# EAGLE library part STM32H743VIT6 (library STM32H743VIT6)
ARM Microcontrollers - MCU High-performance and DSP with DP-FPU, ARM Cortex-M7 MCU with 2MBytes Flash, 1MB RAM, 400 MHz CPU, Art Accelerator, L1 cache, external memory interface, large set of peripherals Source: Datasheet
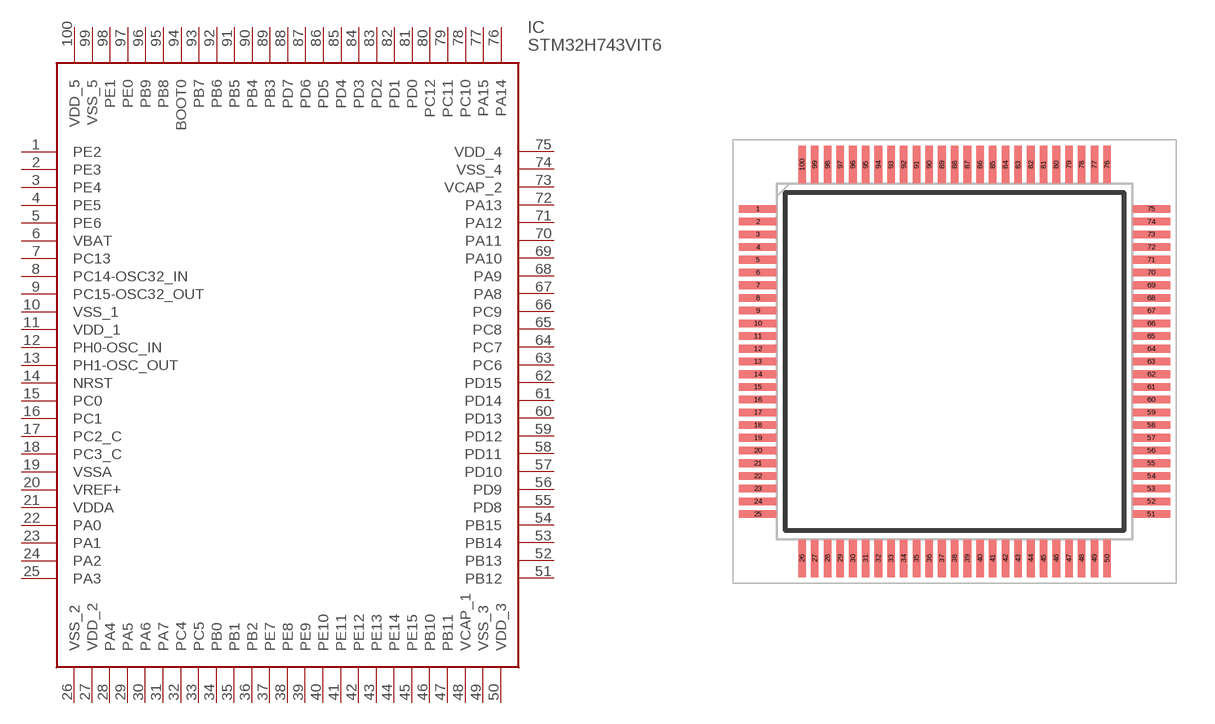
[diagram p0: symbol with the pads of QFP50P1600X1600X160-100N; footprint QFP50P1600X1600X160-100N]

Designator prefix IC

## STM32H743VIT6 (Arrow_Part_Number: STM32H743VIT6; Arrow_Price-Stock: https://www.arrow.com/en/products/stm32h743vit6/stmicroelectronics; Description: ARM Microcontrollers - MCU High-performance and DSP with DP-FPU, ARM Cortex-M7 MCU with 2MBytes Flash, 1MB RAM, 400 MHz CPU, Art Accelerator, L1 cache, external memory interface, large set of peripherals; Height: 1.6mm; Manufacturer_Name: STMicroelectronics; Manufacturer_Part_Number: STM32H743VIT6; Mouser_Part_Number: 511-STM32H743VIT6; Mouser_Price-Stock: https://www.mouser.co.uk/ProductDetail/STMicroelectronics/STM32H743VIT6?qs=FNcb6ahWXRw0Me5k2ZHgWw%3D%3D)  [QFP50P1600X1600X160-100N]
1  PE2
2  PE3
3  PE4
4  PE5
5  PE6
6  VBAT
7  PC13
8  PC14-OSC32_IN
9  PC15-OSC32_OUT
10  VSS_1
11  VDD_1
12  PH0-OSC_IN
13  PH1-OSC_OUT
14  NRST
15  PC0
16  PC1
17  PC2_C
18  PC3_C
19  VSSA
20  VREF+
21  VDDA
22  PA0
23  PA1
24  PA2
25  PA3
26  VSS_2
27  VDD_2
28  PA4
29  PA5
30  PA6
31  PA7
32  PC4
33  PC5
34  PB0
35  PB1
36  PB2
37  PE7
38  PE8
39  PE9
40  PE10
41  PE11
42  PE12
43  PE13
44  PE14
45  PE15
46  PB10
47  PB11
48  VCAP_1
49  VSS_3
50  VDD_3
51  PB12
52  PB13
53  PB14
54  PB15
55  PD8
56  PD9
57  PD10
58  PD11
59  PD12
60  PD13
61  PD14
62  PD15
63  PC6
64  PC7
65  PC8
66  PC9
67  PA8
68  PA9
69  PA10
70  PA11
71  PA12
72  PA13
73  VCAP_2
74  VSS_4
75  VDD_4
76  PA14
77  PA15
78  PC10
79  PC11
80  PC12
81  PD0
82  PD1
83  PD2
84  PD3
85  PD4
86  PD5
87  PD6
88  PD7
89  PB3
90  PB4
91  PB5
92  PB6
93  PB7
94  BOOT0
95  PB8
96  PB9
97  PE0
98  PE1
99  VSS_5
100  VDD_5

## Footprint QFP50P1600X1600X160-100N (pad centres in mm)
LQFP100
smd 1.475 x 0.3: 1 -7.738,6; 2 -7.738,5.5; 3 -7.738,5; 4 -7.738,4.5; 5 -7.738,4; 6 -7.738,3.5; 7 -7.738,3; 8 -7.738,2.5; 9 -7.738,2; 10 -7.738,1.5; 11 -7.738,1; 12 -7.738,0.5; 13 -7.738,0; 14 -7.738,-0.5; 15 -7.738,-1; 16 -7.738,-1.5; 17 -7.738,-2; 18 -7.738,-2.5; 19 -7.738,-3; 20 -7.738,-3.5; 21 -7.738,-4; 22 -7.738,-4.5; 23 -7.738,-5; 24 -7.738,-5.5; 25 -7.738,-6; 51 7.738,-6; 52 7.738,-5.5; 53 7.738,-5; 54 7.738,-4.5; 55 7.738,-4; 56 7.738,-3.5; 57 7.738,-3; 58 7.738,-2.5; 59 7.738,-2; 60 7.738,-1.5; 61 7.738,-1; 62 7.738,-0.5; 63 7.738,0; 64 7.738,0.5; 65 7.738,1; 66 7.738,1.5; 67 7.738,2; 68 7.738,2.5; 69 7.738,3; 70 7.738,3.5; 71 7.738,4; 72 7.738,4.5; 73 7.738,5; 74 7.738,5.5; 75 7.738,6
smd 0.3 x 1.475: 26 -6,-7.738; 27 -5.5,-7.738; 28 -5,-7.738; 29 -4.5,-7.738; 30 -4,-7.738; 31 -3.5,-7.738; 32 -3,-7.738; 33 -2.5,-7.738; 34 -2,-7.738; 35 -1.5,-7.738; 36 -1,-7.738; 37 -0.5,-7.738; 38 0,-7.738; 39 0.5,-7.738; 40 1,-7.738; 41 1.5,-7.738; 42 2,-7.738; 43 2.5,-7.738; 44 3,-7.738; 45 3.5,-7.738; 46 4,-7.738; 47 4.5,-7.738; 48 5,-7.738; 49 5.5,-7.738; 50 6,-7.738; 76 6,7.738; 77 5.5,7.738; 78 5,7.738; 79 4.5,7.738; 80 4,7.738; 81 3.5,7.738; 82 3,7.738; 83 2.5,7.738; 84 2,7.738; 85 1.5,7.738; 86 1,7.738; 87 0.5,7.738; 88 0,7.738; 89 -0.5,7.738; 90 -1,7.738; 91 -1.5,7.738; 92 -2,7.738; 93 -2.5,7.738; 94 -3,7.738; 95 -3.5,7.738; 96 -4,7.738; 97 -4.5,7.738; 98 -5,7.738; 99 -5.5,7.738; 100 -6,7.738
